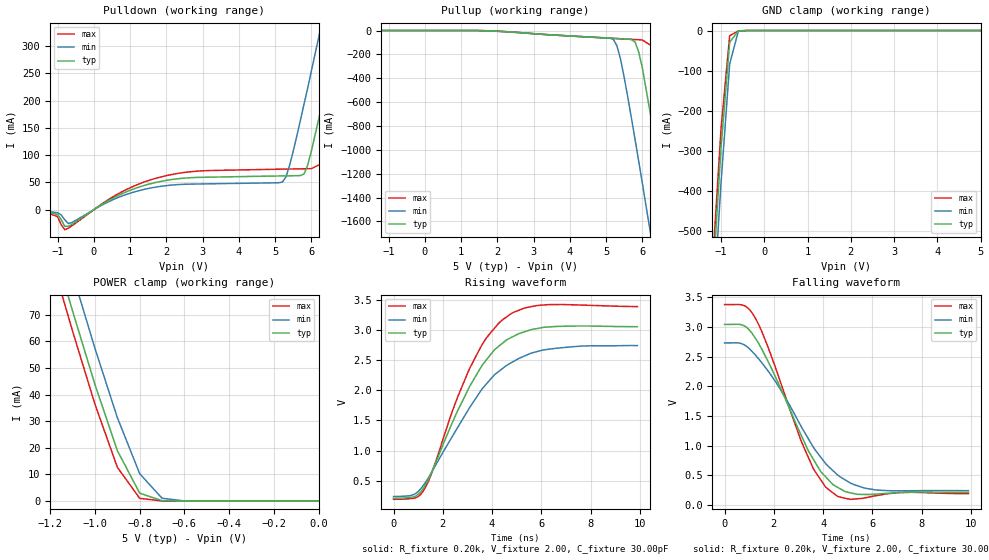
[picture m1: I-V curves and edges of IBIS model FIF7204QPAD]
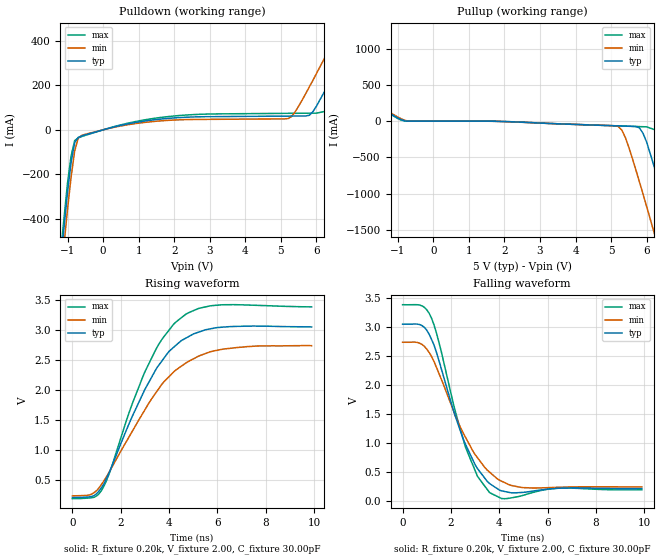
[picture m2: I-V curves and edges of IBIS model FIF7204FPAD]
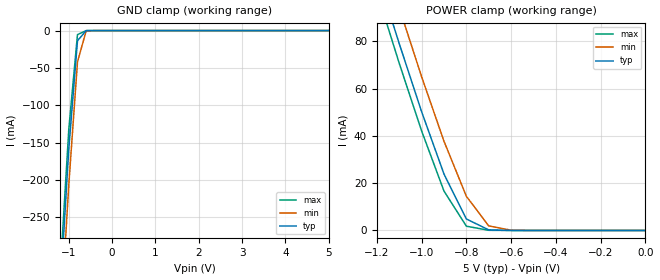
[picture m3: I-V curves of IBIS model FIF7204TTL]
| IBIS file idt7284.ibs created by s2ibis2 version 1.1
| North Carolina State University Electronics Research Laboratory  1995
[IBIS ver]   2.1
[File name]   idt7284.ibs
[File Rev]   1.0
[Date]   07/15/98
[Source]   Integrated Device Technology, Inc.
[Notes]   1. Temperatures: typ=25C, min=70C, max=0C 2. Cemos8_5v
   process. 3. Ramp rates based on 50 ohm load.
[Copyright]   Copyright 1997, Integrated Device Technology, Inc.
|   Component idt7284
[Component]   idt7284
[Manufacturer]   Integrated Device Technology
[Package]
| variable   typ   min   max
R_pkg   0.75   0.60   0.90
L_pkg   8.10nH   8.30nH   9.90nH
C_pkg   0.53pF   0.46pF   0.60pF
[Pin]  signal_name   model_name   R_pin   L_pin   C_pin
1   FFAL   FIF7204FPAD
2   QA0   FIF7204QPAD
3   QA1   FIF7204QPAD
4   QA2   FIF7204QPAD
5   QA3   FIF7204QPAD
6   QA8   FIF7204QPAD
7   GND   GND
8   RAL   FIF7204TTL
9   QA4   FIF7204QPAD
10   QA5   FIF7204QPAD
11   QA6   FIF7204QPAD
12   QA7   FIF7204QPAD
13   XOLHFAL   FIF7204FPAD
14   EFAL   FIF7204FPAD
15   FFBL   FIF7204FPAD
16   QB0   FIF7204QPAD
17   QB1   FIF7204QPAD
18   QB2   FIF7204QPAD
19   QB3   FIF7204QPAD
20   QB8   FIF7204QPAD
21   GND   GND
22   RBL   FIF7204TTL
23   QB4   FIF7204QPAD
24   QB5   FIF7204QPAD
25   QB6   FIF7204QPAD
26   QB7   FIF7204QPAD
27   XOLHFBL   FIF7204FPAD
28   EFBL   FIF7204FPAD
29   RSBL   FIF7204TTL
30   FLRTBL   FIF7204TTL
31   DB7   FIF7204TTL
32   DB6   FIF7204TTL
33   DB5   FIF7204TTL
34   DB4   FIF7204TTL
35   VCC   POWER
36   WBL   FIF7204TTL
37   DB8   FIF7204TTL
38   DB3   FIF7204TTL
39   DB2   FIF7204TTL
40   DB1   FIF7204TTL
41   DB0   FIF7204TTL
42   XIBL   FIF7204TTL
43   RSAL   FIF7204TTL
44   FLRTAL   FIF7204TTL
45   DA7   FIF7204TTL
46   DA6   FIF7204TTL
47   DA5   FIF7204TTL
48   DA4   FIF7204TTL
49   VCC   POWER
50   WAL   FIF7204TTL
51   DA8   FIF7204TTL
52   DA3   FIF7204TTL
53   DA2   FIF7204TTL
54   DA1   FIF7204TTL
55   DA0   FIF7204TTL
56   XIAL   FIF7204TTL
| Models and submodels in the file (3): FIF7204QPAD (3-state), FIF7204FPAD (Output), FIF7204TTL (Input)
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| FIN  FIN   dummy_model
| QIN  QIN   dummy_model
| QOEL QOEL   dummy_model
|   Model FIF7204QPAD
[Model]   FIF7204QPAD
Model_type   3-state
Polarity   Non-Inverting
Enable   Active-Low
Vmeas =  1.500V
C_comp   3.00pF   NA   NA
[Temperature Range]   25.00   70.00   0.000
[Voltage Range]   5.00V   4.50V   5.50V
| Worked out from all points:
|   slope of the pulldown table from 0 to 0.75 V, typ, clamps not added: 26.4 ohm
|   GND clamp passes 1 mA (typ) near -0.58 V on its own axis
|   POWER clamp passes 1 mA (typ) near -0.73 V on its own axis
|   rising waveform, R_fixture 0.20k, V_fixture 2.00, C_fixture 30.00pF: 20-80 % time 2.04ns typ, 2.38ns min, 1.86ns max; typ from 0.212 V to 3.05 V
|   falling waveform, R_fixture 0.20k, V_fixture 2.00, C_fixture 30.00pF: 20-80 % time 1.9ns typ, 2.22ns min, 1.68ns max; typ from 3.04 V to 0.212 V
[Pulldown]
| voltage   I(typ)   I(min)   I(max)
-5V       0A         0A         0A
-1.4V     -3mA       -2mA       -2.6mA
-800mV    -30.42mA   -18.6mA    -36.69mA
1.7V      49.86mA    41.4mA     57.4mA
5.2V      62.01mA    50.61mA    74.43mA
5.4V      62.22mA    81.07mA    74.66mA
5.8V      65.63mA    194mA      75.11mA
6V        107mA      254mA      75.33mA
6.4V      223mA      376mA      88.46mA
6.8V      345mA      500mA      198mA
7.2V      469mA      624mA      320mA
10V       1.346A     1.502A     1.195A
[Pullup]
| voltage   I(typ)   I(min)   I(max)
-5V       0A         0A         0A
1.5V      -479uA     -1.046mA   -164uA
5.2V      -65.7mA    -73.36mA   -65.97mA
5.3V      -67.33mA   -129mA     -67.59mA
5.4V      -68.96mA   -242mA     -69.22mA
5.8V      -96.18mA   -914mA     -75.69mA
6V        -312mA     -1.279A    -78.93mA
6.4V      -1.008A    -2.023A    -157mA
6.8V      -1.75A     -2.776A    -778mA
7.2V      -2.503A    -3.534A    -1.516A
7.6V      -3.262A    -4.295A    -2.268A
10V       -7.849A    -8.885A    -6.849A
[GND_clamp]
| voltage   I(typ)   I(min)   I(max)
-5V       -7.849A    -7.926A    -7.807A
-1.2V     -640mA     -729mA     -591mA
-1V       -293mA     -381mA     -246mA
-800mV    -29.29mA   -83.51mA   -12.91mA
-600mV    -1.086mA   -1.828mA   -995uA
-400mV    -11.7nA    -1.657uA   -4.457nA
5V        50nA       1.239uA    50nA
[POWER_clamp]
| voltage   I(typ)   I(min)   I(max)
-5V       1.28A      1.292A     1.273A
-1.2V     100mA      114mA      92.56mA
-1.1V     71.31mA    85.16mA    63.76mA
-1V       43.75mA    57.31mA    36.34mA
-900mV    18.98mA    31.36mA    12.72mA
-800mV    2.991mA    10.3mA     1.049mA
-700mV    169uA      1.084mA    64.47uA
-600mV    6.517uA    77.91uA    260nA
0V        50nA       45nA       55nA
[Ramp]
| variable   typ   min   max
dV/dt_r   1.00/1.09n   0.85/1.34n   1.15/0.96n
dV/dt_f   1.68/1.86n   1.37/2.24n   1.96/1.60n
R_load = 50.00
[Rising Waveform]
R_fixture = 0.20k
V_fixture = 2.00
C_fixture = 30.00pF
R_dut = 0.75
L_dut = 8.10nH
C_dut = 0.53pF
| time   V(typ)   V(min)   V(max)
0s        212mV      240mV      193mV
900ps     247mV      290mV      219mV
1.3ns     435mV      475mV      393mV
2.5ns     1.568V     1.314V     1.778V
3.1ns     2.071V     1.72V      2.371V
3.7ns     2.468V     2.072V     2.824V
4.4ns     2.772V     2.353V     3.16V
5.3ns     2.968V     2.566V     3.361V
6.1ns     3.044V     2.67V      3.414V
9.9ns     3.054V     2.741V     3.387V
[Falling Waveform]
R_fixture = 0.20k
V_fixture = 2.00
C_fixture = 30.00pF
R_dut = 0.75
L_dut = 8.10nH
C_dut = 0.53pF
| time   V(typ)   V(min)   V(max)
0s        3.045V     2.733V     3.38V
700ps     3.038V     2.719V     3.375V
1.2ns     2.844V     2.553V     3.188V
1.8ns     2.392V     2.241V     2.624V
3.1ns     1.186V     1.331V     1.089V
3.6ns     773mV      977mV      616mV
4.2ns     431mV      655mV      267mV
4.9ns     224mV      421mV      112mV
5.7ns     176mV      283mV      119mV
9.9ns     212mV      241mV      190mV
|   Model FIF7204FPAD
[Model]   FIF7204FPAD
Model_type   Output
Vmeas =  1.500V
C_comp   3.00pF   NA   NA
[Temperature Range]   25.00   70.00   0.000
[Voltage Range]   5.00V   4.50V   5.50V
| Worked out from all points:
|   slope of the pulldown table from 0 to 0.75 V, typ, clamps not added: 26.4 ohm
|   rising waveform, R_fixture 0.20k, V_fixture 2.00, C_fixture 30.00pF: 20-80 % time 2.02ns typ, 2.37ns min, 1.84ns max; typ from 0.212 V to 3.05 V
|   falling waveform, R_fixture 0.20k, V_fixture 2.00, C_fixture 30.00pF: 20-80 % time 1.37ns typ, 1.64ns min, 1.2ns max; typ from 3.04 V to 0.211 V
[Pulldown]
| voltage   I(typ)   I(min)   I(max)
-5V       -7.235A    -7.306A    -7.197A
-1.4V     -927mA     -1.008A    -883mA
-1V       -279mA     -356mA     -239mA
-800mV    -57.48mA   -95.52mA   -48.71mA
-600mV    -27.74mA   -25.09mA   -30.34mA
1.8V      51.31mA    42.46mA    59.24mA
5.2V      62.01mA    50.61mA    74.43mA
5.8V      65.63mA    194mA      75.11mA
6.4V      223mA      376mA      88.46mA
7.2V      469mA      624mA      320mA
7.6V      593mA      749mA      444mA
10V       1.346A     1.502A     1.195A
[Pullup]
| voltage   I(typ)   I(min)   I(max)
-5V       1.28A      1.292A     1.273A
-1.4V     160mA      173mA      152mA
-800mV    2.991mA    10.3mA     1.049mA
5.2V      -65.7mA    -72.45mA   -65.97mA
5.4V      -68.96mA   -225mA     -69.22mA
5.8V      -93.94mA   -843mA     -75.69mA
6V        -289mA     -1.179A    -78.93mA
6.4V      -929mA     -1.865A    -149mA
6.8V      -1.613A    -2.559A    -718mA
7.2V      -2.308A    -3.258A    -1.397A
7.6V      -3.007A    -3.959A    -2.091A
10V       -7.235A    -8.19A     -6.313A
[Ramp]
| variable   typ   min   max
dV/dt_r   1.00/1.11n   0.85/1.33n   1.15/0.93n
dV/dt_f   1.68/0.81n   1.37/0.97n   1.97/0.71n
R_load = 50.00
[Rising Waveform]
R_fixture = 0.20k
V_fixture = 2.00
C_fixture = 30.00pF
R_dut = 0.75
L_dut = 8.10nH
C_dut = 0.53pF
| time   V(typ)   V(min)   V(max)
0s        212mV      240mV      193mV
800ps     230mV      269mV      208mV
1.2ns     374mV      428mV      328mV
1.6ns     702mV      693mV      695mV
3ns       2.013V     1.673V     2.306V
3.6ns     2.43V      2.04V      2.781V
4.3ns     2.753V     2.341V     3.14V
5.2ns     2.963V     2.562V     3.358V
6.2ns     3.049V     2.681V     3.422V
9.9ns     3.053V     2.741V     3.387V
[Falling Waveform]
R_fixture = 0.20k
V_fixture = 2.00
C_fixture = 30.00pF
R_dut = 0.75
L_dut = 8.10nH
C_dut = 0.53pF
| time   V(typ)   V(min)   V(max)
0s        3.045V     2.733V     3.38V
800ps     3.021V     2.696V     3.361V
1.2ns     2.78V      2.487V     3.146V
2.6ns     976mV      1.098V     929mV
3.1ns     555mV      742mV      422mV
3.6ns     298mV      494mV      142mV
4.1ns     171mV      338mV      38.59mV
5ns       146mV      227mV      95.94mV
6.4ns     215mV      233mV      217mV
9.9ns     211mV      240mV      190mV
|   Model FIF7204TTL
[Model]   FIF7204TTL
Model_type   Input
Vinl =  0.000V
Vinh =  3.000V
Vmeas =  1.500V
C_comp   3.00pF   NA   NA
[Temperature Range]   25.00   70.00   0.000
[Voltage Range]   5.00V   4.50V   5.50V
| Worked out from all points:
|   GND clamp passes 1 mA (typ) near -0.61 V on its own axis
|   POWER clamp passes 1 mA (typ) near -0.72 V on its own axis
[GND_clamp]
| voltage   I(typ)   I(min)   I(max)
-5V       -4.391A    -4.433A    -4.368A
-1.2V     -352mA     -401mA     -325mA
-1V       -158mA     -206mA     -132mA
-800mV    -13.64mA   -42.01mA   -5.422mA
-600mV    -95.52uA   -487uA     -19.78uA
5V        50nA       2.529uA    50nA
[POWER_clamp]
| voltage   I(typ)   I(min)   I(max)
-5V       1.33A      1.343A     1.323A
-1.2V     109mA      124mA      101mA
-1.1V     79.07mA    94.22mA    70.74mA
-1V       50.25mA    65.05mA    42.12mA
-900mV    23.87mA    37.74mA    16.67mA
-800mV    4.863mA    14.45mA    1.814mA
-700mV    253uA      1.929mA    79.02uA
-600mV    7.842uA    115uA      476nA
0V        50nA       45nA       55nA
